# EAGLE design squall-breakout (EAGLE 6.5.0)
AUTHOR: Brad Campbell; REV: A; TITLE: Squall Breakout
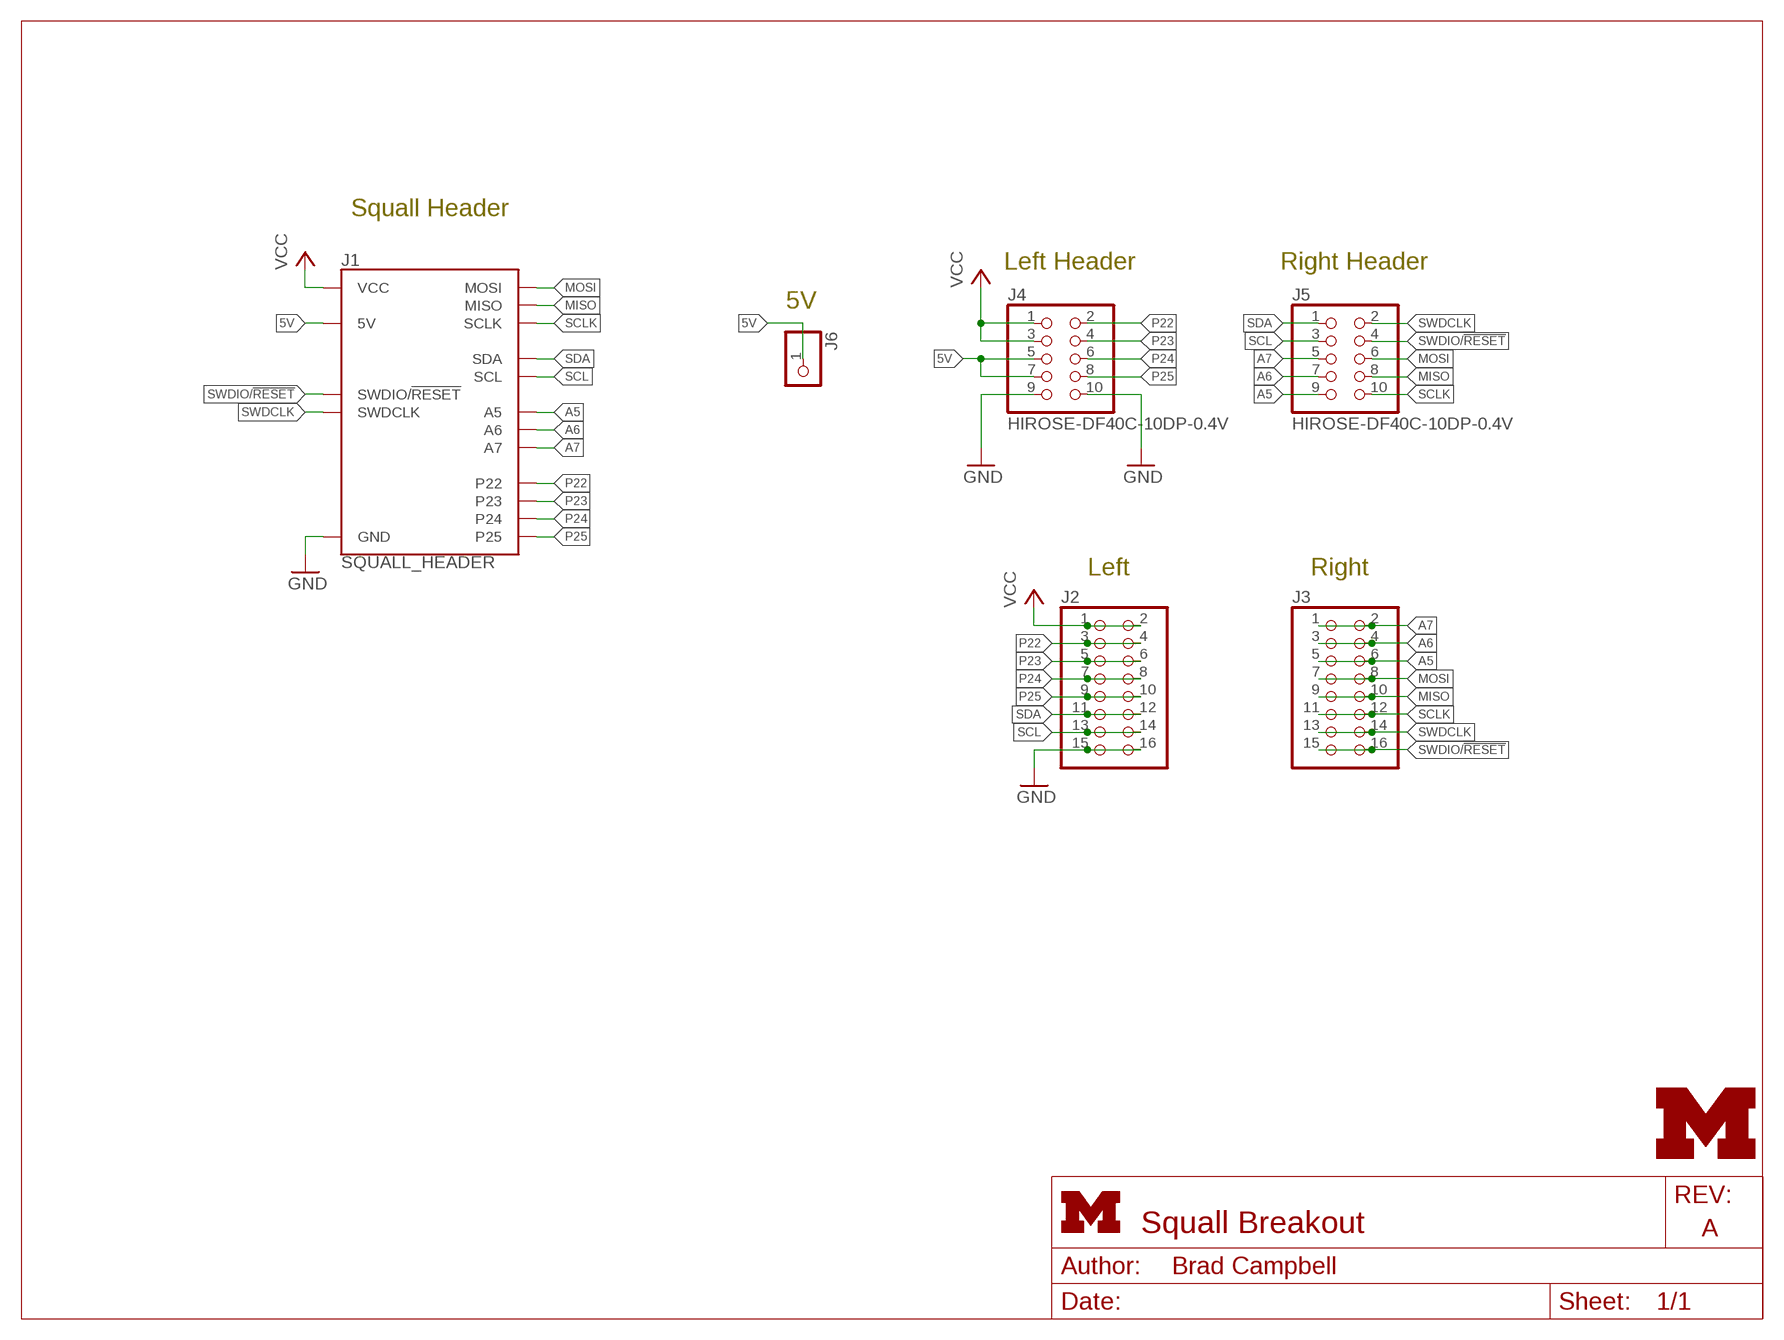
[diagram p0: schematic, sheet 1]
FRAME1 (LETTER_L): HEIGHT: 8.5in; WIDTH: 11in

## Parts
J1  SQUALL_HEADER  [SQUALL_HEADER]
J2  PINHD-2X8  [2X08]
J3  PINHD-2X8  [2X08]
J4  HIROSE-DF40C-10DP-0.4V  [2X5/SMD/0.4MM]
J5  HIROSE-DF40C-10DP-0.4V  [2X5/SMD/0.4MM]
J6  PINHD-1X1  [1X01]
LOGO1  UMICH_SOLID_TINY  [UMICH_SOLID_50MIL]

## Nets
5V: J1.A5(5V) J1.A7(5V) J4.5 J4.7 J6.1
A5: J1.B9(A5) J3.5 J3.6 J5.9
A6: J1.B7(A6) J3.3 J3.4 J5.7
A7: J1.B5(A7) J3.1 J3.2 J5.5
GND: J1.A9(GND) J1.A10(GND) J2.15 J2.16 J4.9 J4.10
MISO: J1.B8(MISO) J3.9 J3.10 J5.8
MOSI: J1.B6(MOSI) J3.7 J3.8 J5.6
P22: J1.A2(P22) J2.3 J2.4 J4.2
P23: J1.A4(P23) J2.5 J2.6 J4.4
P24: J1.A6(P24) J2.7 J2.8 J4.6
P25: J1.A8(P25) J2.9 J2.10 J4.8
SCL: J1.B3(SCL) J2.13 J2.14 J5.3
SCLK: J1.B10(SCLK) J3.11 J3.12 J5.10
SDA: J1.B1(SDA) J2.11 J2.12 J5.1
SWDCLK: J1.B2(SWDCLK) J3.13 J3.14 J5.2
SWDIO/!RESET: J1.B4(SWDIO/!RESET) J3.15 J3.16 J5.4
VCC: J1.A1(VCC) J1.A3(VCC) J2.1 J2.2 J4.1 J4.3

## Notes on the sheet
- Squall Header
- Left Header | Right Header
- 5V
- Left | Right

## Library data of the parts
J1 = squall:SQUALL_HEADER: Header for a sensor board on top of the Squall BLE tag board. Requires two DF40C-10DS-0.4V(51).; DIGIKEY: H11617CT-ND
J2 J3 = pinhead:PINHD-2X8: PIN HEADER
J4 J5 = headers:HIROSE-DF40C-10DP-0.4V: DF40 Series Header - 0.4MM Pitch; DIGIKEY: H11616CT-ND; MOUSER: 798-DF40C10DP0.4V51; NEWARK: 68X2585
J6 = pinhead:PINHD-1X1: PIN HEADER
LOGO1 = logos:UMICH_SOLID

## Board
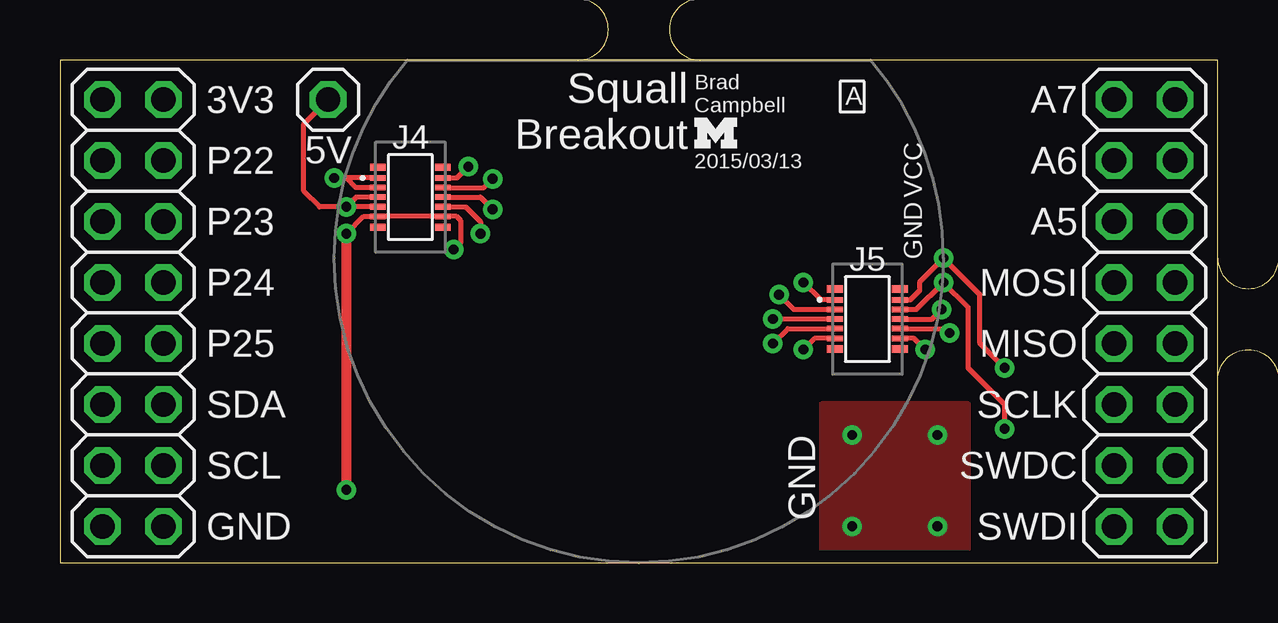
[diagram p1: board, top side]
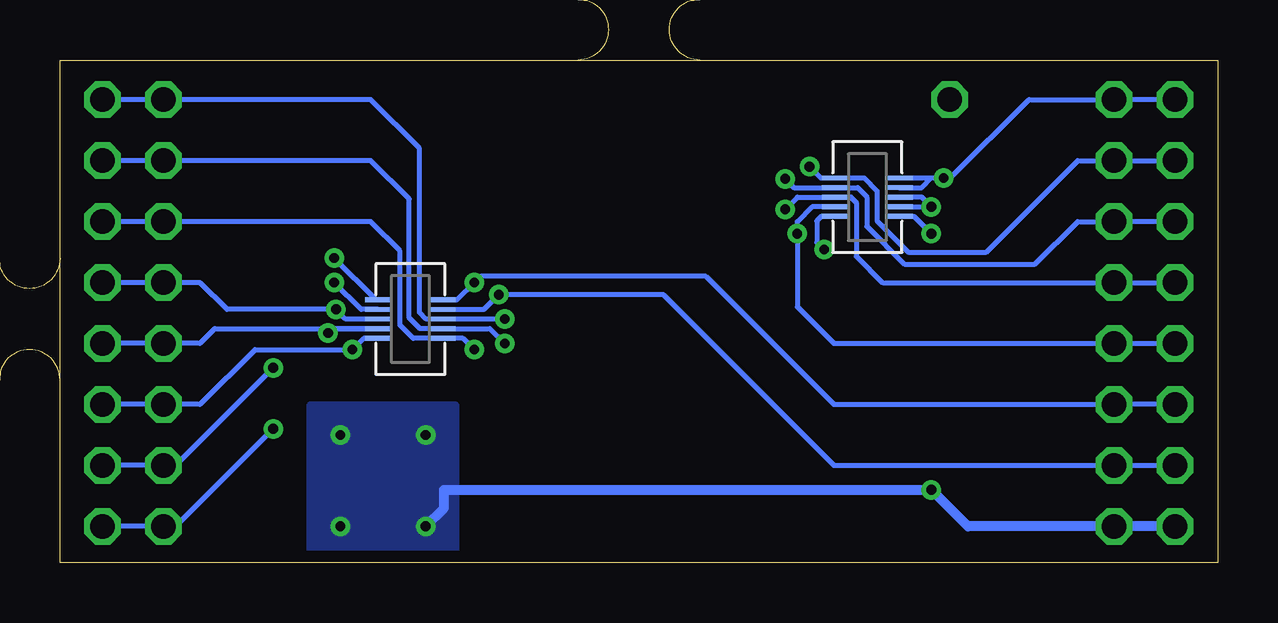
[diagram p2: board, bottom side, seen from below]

Size 48.26 x 20.95 mm. Coordinates in mm from the lower left corner, seen from the top.
Outline: 0,0 48.26,0 48.26,20.95 0,20.95 0,0
Copper layers (1*16): Top 0.0178mm / dielectric 59mil / Bottom 0.0178mm
Design rules "sunstone-2lyr_v1.0.0.3 *": minimum track width 6mil, minimum drill 14mil, track to track 6mil, track to pad 6mil, pad to pad 6mil, via to via 6mil, smd to smd 6mil, copper to edge 20mil, drill to drill 16mil, minimum pad ring 8mil, minimum via ring 8mil, stop-mask expansion 3mil, vias tented up to drill 20mil, thermal gap 10mil
Milling: 10 lines

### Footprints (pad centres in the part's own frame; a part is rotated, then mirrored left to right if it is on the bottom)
SQUALL_HEADER = smd 1.14 x 0.2 bottom: A1 -10.845,3.34; A2 -8.205,3.34; A3 -10.845,2.94; A4 -8.205,2.94; A5 -10.845,2.54; A6 -8.205,2.54; A7 -10.845,2.14; A8 -8.205,2.14; A9 -10.845,1.74; A10 -8.205,1.74; B1 8.205,-1.74; B2 10.845,-1.74; B3 8.205,-2.14; B4 10.845,-2.14; B5 8.205,-2.54; B6 10.845,-2.54; B7 8.205,-2.94; B8 10.845,-2.94; B9 8.205,-3.34; B10 10.845,-3.34
2X08 = drill 1.016 octagon: 1 -8.89,-1.27; 2 -8.89,1.27; 3 -6.35,-1.27; 4 -6.35,1.27; 5 -3.81,-1.27; 6 -3.81,1.27; 7 -1.27,-1.27; 8 -1.27,1.27; 9 1.27,-1.27; 10 1.27,1.27; 11 3.81,-1.27; 12 3.81,1.27; 13 6.35,-1.27; 14 6.35,1.27; 15 8.89,-1.27; 16 8.89,1.27
2X5/SMD/0.4MM = smd 0.66 x 0.23: 1 -1.355,0.8; 2 1.355,0.8; 3 -1.355,0.4; 4 1.355,0.4; 5 -1.355,0; 6 1.355,0; 7 -1.355,-0.4; 8 1.355,-0.4; 9 -1.355,-0.8; 10 1.355,-0.8 | smd 0.66 x 0.3: A -1.355,1.25; B 1.355,1.25; C -1.355,-1.25; D 1.355,-1.25
1X01 = drill 1.016 octagon: 1 0,0

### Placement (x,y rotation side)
J1  24.13,12.7 0 top
J2  3.05,10.41 270 top
J3  45.21,10.41 270 top
J4  14.61,15.24 0 top
J5  33.66,10.16 0 top
J6  11.18,19.3 0 top
LOGO1  27.33,17.91 0 top

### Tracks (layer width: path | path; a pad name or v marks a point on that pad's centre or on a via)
5V  (via drill 0.41)
  Top 0.203: J4.7 v11.94,14.84 | v11.94,14.84 10.81,14.84 10.16,15.49 10.16,18.29 J6.1 | J4.5 12.34,15.24 v11.94,14.84
  Bottom 0.203: J1.A7 v11.94,14.84 12.34,15.24 J1.A5
A5  (via drill 0.41)
  Top 0.203: J5.9 31.46,9.36 v30.99,8.89
  Bottom 0.203: J3.6 J3.5 35.31,14.22 34.09,13.01 34.09,9.91 33.54,9.36 J1.B9 31.46,9.36 v30.99,8.89
A6  (via drill 0.41)
  Top 0.203: v29.72,9.14 30.33,9.76 J5.7
  Bottom 0.203: J3.4 J3.3 35.31,16.76 33.71,15.16 33.71,10.21 33.26,9.76 J1.B7 30.33,9.76 v29.72,9.14
A7  (via drill 0.41)
  Top 0.203: J5.5 v29.72,10.16
  Bottom 0.203: J3.2 J3.1 35.31,19.3 33.27,17.27 33.27,10.44 32.99,10.16 J1.B5 v29.72,10.16
GND  (via drill 0.41)
  Top 0.203: v11.94,13.72 12.66,14.44 J4.9 J4.10 16.52,14.44 16.71,14.25 16.71,13.36 v16.41,13.06
  Top 0.406: v11.94,3.05 v11.94,13.72
  Bottom 0.203: J1.A9 12.66,14.44 v11.94,13.72 | J1.A10 16.52,14.44 16.71,14.25 16.71,13.36 v16.41,13.06
  Bottom 0.406: J2.15 J2.16 10.41,1.52 v11.94,3.05 32.26,3.05 32.26,2.29 v33.02,1.52
  other vias: 33.02,5.33 36.58,5.33 36.58,1.52
  pour Bottom: 37.85,0.51 37.85,6.6 31.75,6.6 31.75,0.51
  pour Top: 37.85,0.51 37.85,6.6 31.75,6.6 31.75,0.51
MISO  (via drill 0.41)
  Top 0.203: J5.8 36.9,9.76 v37.08,9.58
  Bottom 0.203: J3.10 J3.9 42.42,9.14 41.8,9.76 J1.B8 36.9,9.76 v37.08,9.58
MOSI  (via drill 0.41)
  Top 0.203: J5.6 36.35,10.16 v36.75,10.57
  Bottom 0.203: J3.8 J3.7 42.42,11.68 41.3,10.57 v36.75,10.57 36.35,10.16 J1.B6
P22  (via drill 0.41)
  Top 0.203: J4.2 16.55,16.04 v17.02,16.51
  Bottom 0.203: J2.3 J2.4 5.84,16.76 9.65,12.95 12.9,12.95 14.2,14.25 14.2,15.49 14.74,16.04 J1.A2 16.55,16.04 v17.02,16.51
P23  (via drill 0.41)
  Top 0.203: J4.4 17.67,15.64 v18.03,16
  Bottom 0.203: J2.5 J2.6 5.84,14.22 7.62,12.45 13.06,12.45 14.63,14.02 14.63,15.27 15.01,15.64 J1.A4 17.67,15.64 v18.03,16
P24  (via drill 0.41)
  Top 0.203: J4.6 17.53,15.24 v18.03,14.73
  Bottom 0.203: J2.7 J2.8 13.97,11.68 15.06,12.78 15.06,15.01 15.29,15.24 J1.A6 17.53,15.24 v18.03,14.73
P25  (via drill 0.41)
  Top 0.203: J4.8 16.91,14.84 17.53,14.22 v17.53,13.72
  Bottom 0.203: J1.A8 16.91,14.84 17.53,14.22 v17.53,13.72 17.53,10.67 16,9.14 J2.10 J2.9
SCL  (via drill 0.41)
  Top 0.203: v29.97,11.18 30.59,10.56 J5.3
  Bottom 0.203: J2.13 J2.14 16,4.06 23.11,11.18 v29.97,11.18 30.59,10.56 J1.B3
SCLK  (via drill 0.41)
  Top 0.203: v36.07,8.89 35.6,9.36 J5.10
  Bottom 0.203: J3.12 J3.11 42.42,6.6 40.13,8.89 v36.07,8.89 35.6,9.36 J1.B10
SDA  (via drill 0.41)
  Top 0.203: J5.1 31.71,10.96 v30.99,11.68
  Bottom 0.203: J1.B1 31.71,10.96 v30.99,11.68 30.73,11.94 21.34,11.94 16,6.6 J2.12 J2.11
SWDCLK  (via drill 0.41)
  Top 0.203: v39.37,8.13 38.35,9.14 38.35,11.18 v36.83,12.7 35.84,11.71 35.84,11.35 35.45,10.96 J5.2
  Bottom 0.203: J3.14 J3.13 43.43,4.06 v39.37,8.13 | J1.B2 35.09,10.96 v36.83,12.7
SWDIO/!RESET  (via drill 0.41)
  Top 0.203: v39.37,5.59 39.37,6.6 37.85,8.13 37.85,10.67 v36.83,11.68 35.71,10.56 J5.4
  Bottom 0.203: J1.B4 35.71,10.56 v36.83,11.68 | J3.16 J3.15 43.43,1.52 v39.37,5.59
VCC  (via drill 0.41)
  Top 0.203: J4.1 v11.43,16.04 11.94,16.04 12.34,15.64 J4.3
  Bottom 0.203: J1.A1 11.94,16.04 | 11.94,16.04 v11.43,16.04 11.14,16.04 7.87,19.3 J2.2 J2.1 | J1.A3 12.34,15.64 11.94,16.04

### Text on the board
tPlace: 3V3 | Brad / Campbell | A | A7 | 5V | P22 | Squall / Breakout | A6 | 2015/03/13 | VCC | P23 | GND | A5 | P24 | MOSI | P25 | MISO | SDA | SCLK | SCL | GND | SWDC | GND | SWDI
